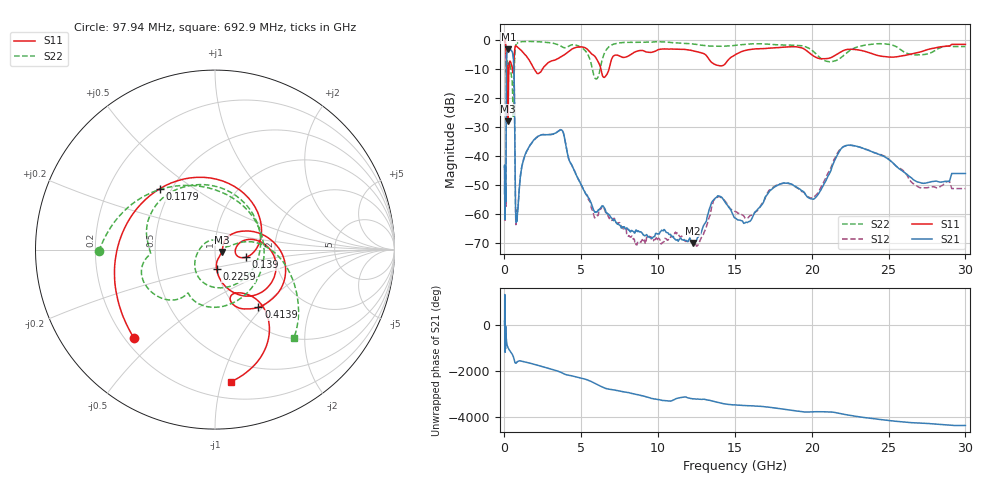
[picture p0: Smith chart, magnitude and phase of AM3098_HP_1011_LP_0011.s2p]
! Date/Time: Thu, Feb 28, 2019 8:43 AM
! Network Analyzer: Agilent Technologies E8364B Rev: A.07.50.67
! Sweep from 0.010 to 30.000 GHz, 1601 Points, Sweep Type: LOG
! Power Supply: 5.022 V, 0.002 A
# Hz S DB R 50
!freq MagS11 AngS11 MagS21 AngS21 MagS12 AngS12 MagS22 AngS22
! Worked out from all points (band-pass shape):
!   1601 points, 10 MHz to 30 GHz, reference 50 ohm
!   highest |S21| = -3.42 dB at 252.2 MHz (marker M1); lowest = -69.8 dB at 12.25 GHz (marker M2)
!   |S21| within 3 dB of the highest: 136.7 MHz to 581.5 MHz (444.8 MHz wide, 124 % of centre)
!   lowest |S11| = -28.1 dB at 239.9 MHz (marker M3), VSWR 1.08, Z = 53.8 - j1.4 ohm
!   |S11| at or under -10 dB: 200.1 MHz to 292.7 MHz (92.59 MHz wide, 37.6 % of centre); 1.92 GHz to 2.495 GHz (574.9 MHz wide, 26 % of centre); 6.271 GHz to 6.815 GHz (544.3 MHz wide, 8.32 % of centre)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
!   |S22| runs from -26.4 to -0.5 dB; largest |S21 - S12| = 0.013
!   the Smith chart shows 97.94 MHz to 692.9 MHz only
!   S11 on the Smith chart (normalised r, x): 97.94 MHz: 0.24, -0.42; 117.9 MHz: 0.43, +0.37; 139 MHz: 1.41, -0.12; 225.9 MHz: 0.99, -0.22; 413.9 MHz: 1.23, -0.95; 692.9 MHz: 0.33, -1.07
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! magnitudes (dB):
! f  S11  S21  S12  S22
! 10 MHz  -0.3  -43.9  -43.0  -0.5
! 38.04 MHz  -0.4  -60.6  -62.4  -0.8
! 97.94 MHz  -3.5  -52.5  -49.8  -3.8
! 117.9 MHz  -6.8  -20.6  -20.7  -10.8
! 139 MHz  -15.0  -5.9  -5.9  -10.6
! 144.7 MHz  -18.3  -5.2  -5.1  -10.9
! 187.7 MHz  -8.8  -4.0  -4.0  -7.2
! 225.9 MHz  -19.3  -3.5  -3.5  -8.7
! 239.9 MHz  -28.1  -3.4  -3.4  -8.9
! 252.2 MHz  -21.4  -3.4  -3.4  -8.8
! 413.9 MHz  -7.9  -3.6  -3.6  -11.0
! 550.5 MHz  -11.5  -5.1  -5.1  -24.3
! 630.1 MHz  -6.1  -12.9  -12.9  -13.6
! 692.9 MHz  -2.6  -45.2  -45.3  -3.6
! 797.2 MHz  -2.4  -62.4  -58.8  -1.4
! 2.084 GHz  -11.4  -33.6  -33.7  -0.7
! 3.723 GHz  -5.8  -31.1  -31.0  -2.4
! 5.959 GHz  -6.4  -59.2  -60.7  -13.6
! 7.926 GHz  -6.0  -64.8  -65.3  -1.0
! 12.25 GHz  -3.8  -69.8  -69.7  -1.5
! 22.56 GHz  -3.3  -36.3  -36.3  -3.5
! 30 GHz  -1.7  -46.0  -51.2  -2.4
